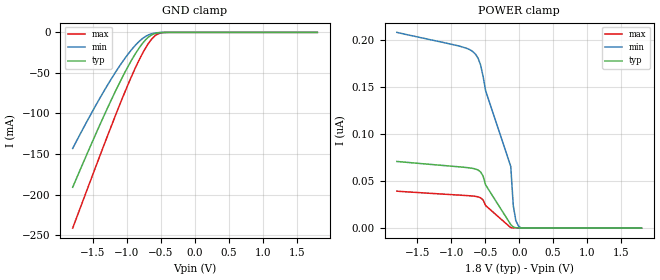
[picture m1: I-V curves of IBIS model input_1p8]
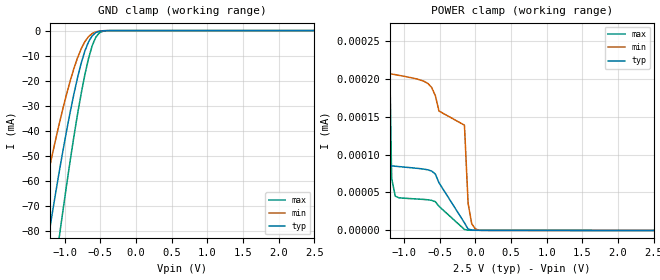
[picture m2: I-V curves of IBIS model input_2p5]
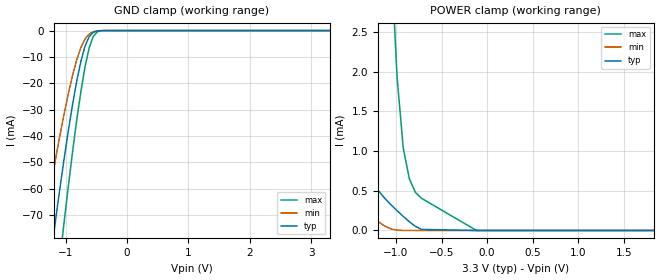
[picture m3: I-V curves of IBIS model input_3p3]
|Texas Instruments Incorporated
| 8-Bit Dual-Supply Bus Transceiver With Configurable Voltage Translation and
| 3-State Outputs
[IBIS Ver]   4.1
[File name]   txv0108.ibs
[Date]   12/05/2023
[File Rev]   1.0
[Source]
| Texas Instruments Incorporated.
| Analog-eLab Design Center, HPA
| 12500 TI Blvd
| Dallas, TX -75243
[Notes]
| Rev 1.0: 12/05/2023
| - Initial release
[Disclaimer]
| This model is designed as an aid for customers of Texas Instruments.
| TI and its licensors and suppliers make no warranties, either expressed
| or implied, with respect to this  model, including the warranties of
| merchantability or fitness for a particular purpose. The model is
| provided solely on an "as is" basis. The entire risk as to its quality
| and performance is with the customer.
[Copyright]
(C) Copyright 2017 Texas Instruments Incorporated.All rights reserved.
|   TXV0108RGY
| Marketing part#   Digital Voltage Range   Package-type   #pins
| TXV0108RGY   1.8V-3.6V   VQFN   24
[Component]   TXV0108RGY
[Manufacturer]  TI
[Package]   |24 VQFN - RGY package
|   typ   min   max
R_pkg   3.700e-02   2.500e-02   5.300e-02
L_pkg   8.060e-10   5.310e-10   1.139e-09
C_pkg   1.880e-13   5.700e-14   3.100e-13
[Pin]  signal_name   model_name   R_pin   L_pin   C_pin
1   VCCA   POWER   4.700e-02   1.028e-09   3.100e-13
2   DIR   input   5.300e-02   1.139e-09   2.800e-13
3   A1   io   3.400e-02   7.350e-10   2.480e-13
4   A2   io   3.300e-02   7.260e-10   2.460e-13
5   A3   io   3.200e-02   6.830e-10   2.620e-13
6   A4   io   3.000e-02   6.550e-10   2.410e-13
7   A5   io   3.000e-02   6.580e-10   2.400e-13
8   A6   io   3.100e-02   6.770e-10   2.330e-13
9   A7   io   3.500e-02   7.590e-10   2.490e-13
10   A8   io   3.700e-02   7.990e-10   2.540e-13
11   GND   GND   4.500e-02   9.840e-10   2.710e-13
12   GND   GND   4.500e-02   9.870e-10   2.580e-13
13   GND   GND   4.100e-02   8.860e-10   2.340e-13
14   B8   io   4.700e-02   1.014e-09   2.510e-13
15   B7   io   3.600e-02   7.740e-10   2.390e-13
16   B6   io   3.600e-02   7.870e-10   2.540e-13
17   B5   io   3.200e-02   7.070e-10   2.350e-13
18   B4   io   2.900e-02   6.430e-10   2.300e-13
19   B3   io   3.000e-02   6.450e-10   2.300e-13
20   B2   io   3.300e-02   7.100e-10   2.360e-13
21   B1   io   3.800e-02   8.150e-10   2.570e-13
22   NOE   input   3.600e-02   7.750e-10   2.390e-13
23   VCCB   POWER   4.700e-02   1.015e-09   2.510e-13
24   VCCB   POWER   4.100e-02   8.850e-10   2.360e-13
|   TXV0108RGY
| Marketing part#   Digital Voltage Range   Package-type   #pins
| TXV0108RGY   1.8V-3.6V   VQFN   24
[Model Selector] input
input_1p8   1.8V   digital Input
input_2p5   2.5V   digital Input
input_3p3   3.3V   digital Input
[Model Selector] io
io_1p8   1.8V   digital I/O
io_2p5   2.5V   digital I/O
io_3p3   3.3V   digital I/O
| Models and submodels in the file (6): input_1p8 (Input), input_2p5 (Input), input_3p3 (Input), io_1p8 (I/O), io_2p5 (I/O), io_3p3 (I/O)
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|   input_1p8 Model
[Model]   input_1p8
Model_type   Input
Vinl =  0.540V
Vinh =  1.260V
|   typ   min   max
C_comp   1.986pF   1.912pF   2.111pF
| Where Nom  PVT is Nominal Process, 1.8V,  27C
|   Fast PVT is Strong Process,  1.95V, -40C
|   Slow PVT is Weak Process,   1.65V, 125C
[Voltage Range]   1.8   1.65   1.95
|Junction Temperature
[Temperature Range]   27   125   -40
[Power Clamp Reference]   1.8   1.65   1.95
[GND Clamp Reference]   0   0   0
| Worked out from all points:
|   GND clamp passes 1 mA (typ) near -0.57 V on its own axis
[GND Clamp]
|Voltage   I(typ)   I(min)   I(max)
-1.8V     -191mA     -143.1mA   -241.4mA
-1.578V   -147.8mA   -107.9mA   -191.8mA
-1.356V   -105.8mA   -74.75mA   -142.6mA
-1.171V   -72.59mA   -49.3mA    -102.6mA
-986mV    -42.13mA   -26.9mA    -64.4mA
-875mV    -26.05mA   -15.67mA   -43.28mA
-764mV    -12.71mA   -7.063mA   -24.62mA
-653mV    -3.853mA   -2.076mA   -9.887mA
-579mV    -1.121mA   -675.7uA   -3.576mA
-505mV    -223.2uA   -170.7uA   -768.7uA
-394mV    -11.53uA   -14.74uA   -30.66uA
1.8V      0A         0A         0A
[POWER Clamp]
|Voltage   I(typ)   I(min)   I(max)
-1.8V     70.75nA    207.7nA    39.26nA
-790mV    64.4nA     191.2nA    34.62nA
-679mV    63.35nA    187.1nA    34.01nA
-605mV    61.67nA    180.3nA    33.2nA
-568mV    59.62nA    173.1nA    32.21nA
-531mV    55.25nA    161nA      29.88nA
-494mV    45.84nA    145.8nA    23.95nA
-124mV    3.805nA    65.43nA    485.7pA
-87mV     1.147nA    23.84nA    235.2pA
-50mV     439pA      8.249nA    184.2pA
-13mV     246.6pA    2.405nA    165pA
1.8V      0A         0A         0A
|   input_2p5 Model
[Model]   input_2p5
Model_type   Input
Vinl = 0.75
Vinh = 1.75
|   typ   min   max
C_comp   1.985pF   1.882pF   2.077pF
| Where Nom  PVT is Nominal Process, 2.5V, 27C
|   Fast PVT is Strong Process,  2.70V, -40C
|   Slow PVT is Weak Process,   2.25, 125C
[Voltage Range]   2.5   2.25   2.75
|Junction Temperature
[Temperature Range]   27   150   -40
[Power Clamp Reference]   2.50   2.25   2.70
[GND Clamp Reference]   0   0   0
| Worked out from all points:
|   GND clamp passes 1 mA (typ) near -0.57 V on its own axis
|   POWER clamp passes 1 mA (typ) near -2.11 V on its own axis
[GND Clamp]
|Voltage   I(typ)   I(min)   I(max)
-2.092V   -248.6mA   -191.1mA   -306.3mA
-1.429V   -119.5mA   -85.39mA   -158.7mA
-1.378V   -109.9mA   -77.92mA   -147.5mA
-1.225V   -82.07mA   -56.47mA   -114.1mA
-1.174V   -73.11mA   -49.69mA   -103.2mA
-1.072V   -55.84mA   -36.85mA   -81.8mA
-817mV    -18.65mA   -10.78mA   -33.14mA
-715mV    -8.118mA   -4.382mA   -17.51mA
-613mV    -2.08mA    -1.169mA   -6.039mA
-511mV    -257.4uA   -192.5uA   -888.4uA
-409mV    -17.82uA   -20.92uA   -50.46uA
2.5V      0A         0A         0A
[POWER_clamp]
|Voltage   I(typ)   I(min)   I(max)
-2.5V     9.06mA     1.505mA    24mA
-1.631V   89.37uA    412nA      361.9uA
-1.427V   634.6nA    210.9nA    115.9uA
-1.325V   97.17nA    208.6nA    22.38uA
-1.223V   85.67nA    206.8nA    356.7nA
-1.172V   85.03nA    205.9nA    68.45nA
-1.121V   84.55nA    205.1nA    45.15nA
-560mV    74.27nA    177.6nA    37.88nA
-152mV    10.06nA    138.6nA    1.335nA
-101mV    1.901nA    35.68nA    364.7pA
1mV       333.1pA    1.981nA    228.7pA
2.5V      0A         0A         0A
|   input_3p3 Model
[Model]   input_3p3
Model_type   Input
Vinl =  0.500V
Vinh =  2.310V
|   typ   min   max
C_comp   1.956pF   1.864pF   1.998pF
| Where Nom  PVT is Nominal Process, 3.3V, 27C
|   Fast PVT is Strong Process,  3.6V, -40C
|   Slow PVT is Weak Process,   3.0V, 130C
[Voltage Range]   3.3   3   3.6
|Junction Temperature
[Temperature Range]   27   125   -40
[Power Clamp Reference]   3.3   3   3.6
[GND Clamp Reference]   0   0   0
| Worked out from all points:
|   GND clamp passes 1 mA (typ) near -0.57 V on its own axis
|   POWER clamp passes 1 mA (typ) near -1.32 V on its own axis
[GND Clamp]
|Voltage   I(typ)   I(min)   I(max)
-2.161V   -262.3mA   -202.7mA   -322.1mA
-1.357V   -106mA     -74.89mA   -142.8mA
-1.223V   -81.71mA   -56.2mA    -113.7mA
-1.156V   -69.99mA   -47.35mA   -99.38mA
-1.089V   -58.65mA   -38.91mA   -85.32mA
-1.022V   -47.76mA   -30.95mA   -71.6mA
-821mV    -19.13mA   -11.09mA   -33.81mA
-687mV    -5.965mA   -3.194mA   -13.85mA
-620mV    -2.337mA   -1.299mA   -6.642mA
-553mV    -661uA     -428.6uA   -2.22mA
-419mV    -23.68uA   -26.36uA   -69.53uA
3.3V      0A         0A         0A
[POWER_clamp]
|Voltage   I(typ)   I(min)   I(max)
-2.395V   12.55mA    3.763mA    27.8mA
-2.06V    10.25mA    2.495mA    24.28mA
-1.591V   5.721mA    630.5uA    16.83mA
-1.457V   3.172mA    377.4uA    13.63mA
-1.323V   1.023mA    231.1uA    10.42mA
-1.122V   403uA      55.42uA    5.418mA
-1.055V   324.2uA    19.6uA     3.488mA
-921mV    178uA      813.6nA    1.046mA
-854mV    110.8uA    273.9nA    652.3uA
-720mV    13.42uA    181.7nA    405.2uA
-117mV    3.335nA    55.92nA    606.8pA
1.826V    63.87pA    0A         113.5pA
